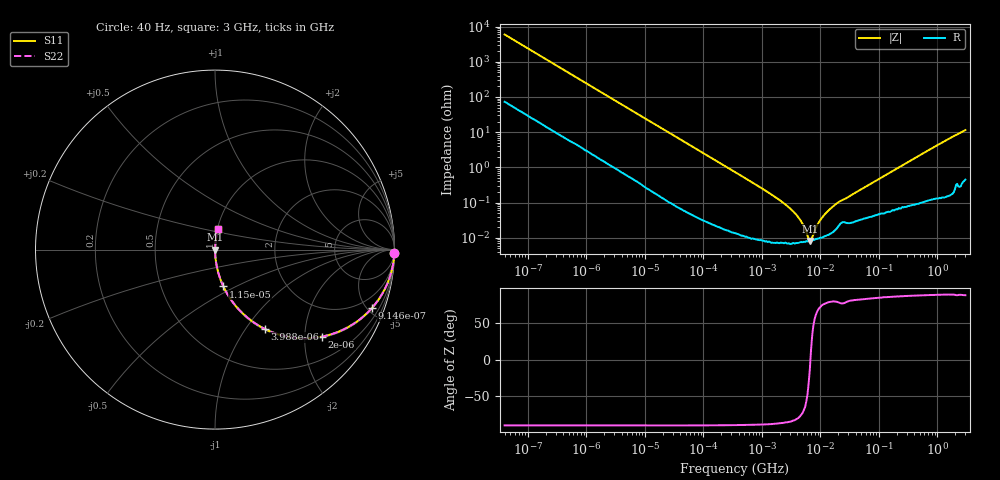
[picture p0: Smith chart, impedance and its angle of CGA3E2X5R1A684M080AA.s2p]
! S-parameter Generated by TDK Corporation
! Copyright(C) 2015 TDK Corporation.
! All Rights Reserved.
! TDK P/N: CGA3E2X5R1A684M080AA (Multilayer Ceramic Chip Capacitors)
! Property: C=680nF
! Size(LxWxT): 1.6x0.8x0.8mm, 0.063x0.031x0.031inches
! Model Type: s2p (Touchstone File Format Version 1.0)
! Frequency: DC=Yes Start=0.00004MHz Stop=3000MHz 396points Log-sweep
! Note: This model was converted from impedance.
! Model Generated on Jun. 23, 2015
! Hash(MD5):
! Port Assignments:
!  1 ---| |--- 2
! Applicable Conditions:
!  Temperature = 25 degC
!  DC Bias Voltage = 0 V
!  Small Signal Operation
! Terms and conditions regarding TDK Simulation Models
! (1)This simulation model is being provided solely for informational purposes. Please refer to the specifications of the products in terms of detailed characteristics of such products.
! (2)In no event shall TDK Corporation of any of its subsidiaries be liable for any loss or damage arising, directly or indirectly,
!  From any information contained in this simulation model, including, but not limited to loss or damages arising from any inaccuracies, omissions or errors in connection with such information.
! (3)Any and all copyrights on this simulation model are owned by TDK Corporation.
!  Duplication or redistribution of this simulation model without prior written permission from TDK Corporation is prohibited.
! (4)This simulation model is subject to any modification or change without any prior notice.
! (5)Neither TDK Corporation nor any of its subsidiaries shall make any warranty, express or implied,
!  Including but not limited to the correctness, implied warranties of merchantability and fitness for a particular purpose with respect to this simulation models.
! (6)The use of this simulation model shall be deemed to have consented to the terms and conditions hereof.
# MHz S MA R 50
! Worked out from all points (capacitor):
!   395 points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, 40 Hz to 3 GHz, reference 50 ohm
!   read as one part in series: C = 668 nF near 41.88 Hz
!   lowest |Z| = 8.14 mohm at 6.589 MHz (marker M1)
!   series resonance near 6.736 MHz, so ESL is about 840 pH
!   S11 on the Smith chart (normalised r, x): 40 Hz: open; 914.6 Hz: 1.06, -5.31; 2 kHz: 1.03, -2.44; 3.988 kHz: 1.01, -1.23; 11.5 kHz: 1.00, -0.43; 3 GHz: 1.01, +0.23
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4e-05  0.9997 -1.0  0.01677 88.3  0.01677 88.3  0.9997 -1.0
0.0002407527  0.9938 -5.7  0.0994 83.6  0.0994 83.6  0.9938 -5.7
0.000834128  0.942 -18.9  0.324 70.4  0.324 70.4  0.942 -18.9
0.0009145504  0.9321 -20.6  0.3512 68.8  0.3512 68.8  0.9321 -20.6
0.001999837  0.7689 -39.1  0.6302 50.3  0.6302 50.3  0.7689 -39.1
0.003988472  0.5212 -57.9  0.8474 31.4  0.8474 31.4  0.5212 -57.9
0.006617114  0.3477 -69.0  0.9335 20.3  0.9335 20.3  0.3477 -69.0
0.01149524  0.2105 -77.2  0.9753 12.1  0.9753 12.1  0.2105 -77.2
0.01739424  0.1417 -81.2  0.9884 8.1  0.9884 8.1  0.1417 -81.2
0.05496573  0.04591 -86.7  0.9984 2.6  0.9984 2.6  0.04591 -86.7
0.3464102  0.007389 -88.5  0.9998 0.4  0.9998 0.4  0.007389 -88.5
1.581893  0.001549 -87.3  0.9999 0.1  0.9999 0.1  0.001549 -87.3
3.013016  0.0006898 -84.4  0.9999 0.0  0.9999 0.0  0.0006898 -84.4
4.5592  0.0003155 -76.1  0.9999 0.0  0.9999 0.0  0.0003155 -76.1
6.292177  9.273e-05 -31.5  0.9999 0.0  0.9999 0.0  9.273e-05 -31.5
6.588528  8.136e-05 -12.9  0.9999 0.0  0.9999 0.0  8.136e-05 -12.9
7.22376  0.0001021 32.8  0.9999 -0.0  0.9999 -0.0  0.0001021 32.8
8.293268  0.000187 60.4  0.9999 -0.0  0.9999 -0.0  0.000187 60.4
9.969551  0.0003233 71.7  0.9999 -0.0  0.9999 -0.0  0.0003233 71.7
16.54008  0.0007914 79.3  0.9999 -0.0  0.9999 -0.0  0.0007914 79.3
150.6385  0.006973 85.1  0.9994 -0.4  0.9994 -0.4  0.006973 85.1
3000  0.1137 81.2  0.9891 -6.5  0.9891 -6.5  0.1137 81.2
